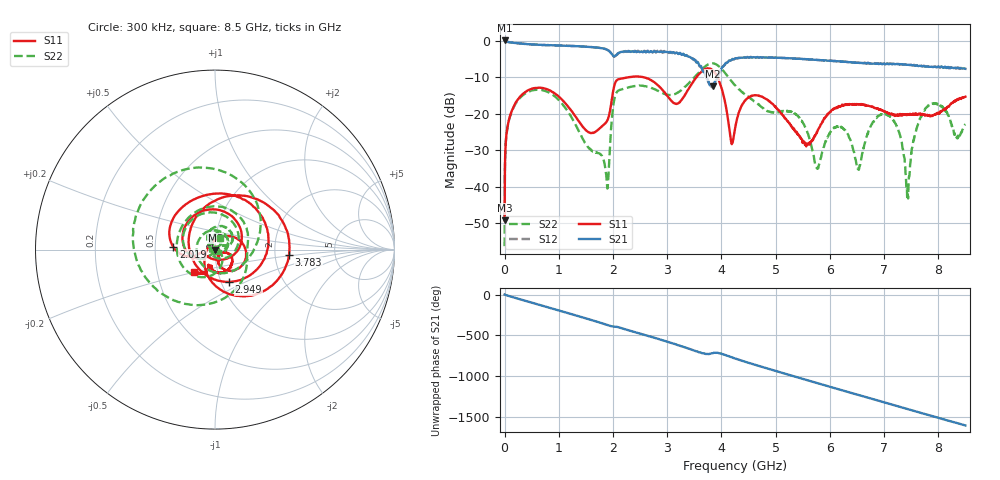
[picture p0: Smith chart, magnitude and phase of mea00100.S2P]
!Agilent Technologies,E5071B,MY42402595,A.08.01
!Date: Tue Jan 02 09:49:13 2001
!Data & Calibration Information:
!Freq	S11:SOLT2(ON)	S21:SOLT2(ON)	S12:SOLT2(ON)	S22:SOLT2(ON)
# Hz S dB R 50
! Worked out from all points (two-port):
!   1601 points, 300 kHz to 8.5 GHz, reference 50 ohm
!   highest |S21| = 0.03 dB at 300 kHz (marker M1); lowest = -12.5 dB at 3.841 GHz (marker M2)
!   |S21| within 3 dB of the highest: start of sweep to 1.937 GHz; 2.228 GHz to 2.254 GHz (25.67 MHz wide, 1.15 % of centre)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
!   lowest |S11| = -49.2 dB at 300 kHz (marker M3), VSWR 1.01, Z = 50.2 - j0.273 ohm
!   |S11| at or under -10 dB: start of sweep to 2.312 GHz; 2.55 GHz to 3.542 GHz (992 MHz wide, 32.6 % of centre); 3.925 GHz to end of sweep
!   |S22| runs from -56.3 to -6.2 dB; largest |S21 - S12| = 0.028
!   S11 on the Smith chart (normalised r, x): 300 kHz: 1.00, -0.01; 2.019 GHz: 0.62, +0.02; 2.949 GHz: 1.09, -0.41; 3.783 GHz: 2.40, -0.16; 8.5 GHz: 0.77, -0.20
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300000  -49.24 -52.1  0.03 0.2  0.00 -0.3  -56.32 -118.4
4.811081e7  -24.21 -137.5  -0.34 -11.0  -0.36 -11.1  -24.28 -137.5
1.490448e8  -18.68 -155.8  -0.58 -31.1  -0.59 -31.1  -18.84 -154.7
4.837204e8  -13.32 134.9  -1.03 -95.7  -1.05 -95.6  -13.77 140.8
8.5027e8  -13.79 59.2  -1.26 -165.2  -1.29 -165.2  -14.49 64.1
1.418687e9  -23.16 -54.0  -1.61 84.7  -1.61 84.7  -26.21 -75.5
1.886171e9  -22.13 -168.3  -2.49 -9.9  -2.49 -10.3  -38.99 106.3
2.018979e9  -12.64 176.2  -4.27 -30.3  -4.43 -30.7  -16.47 -101.2
2.428027e9  -9.83 53.6  -3.06 -104.3  -3.16 -103.9  -12.38 103.4
2.837075e9  -12.33 -36.3  -3.03 176.8  -3.03 175.1  -13.83 26.0
2.948633e9  -14.16 -66.7  -3.10 154.9  -2.92 153.7  -14.63 10.6
3.782666e9  -7.67 -3.9  -12.16 -5.1  -11.76 -4.1  -6.37 153.2
3.841102e9  -8.19 -24.6  -12.54 3.3  -12.16 5.8  -6.24 129.7
4.25015e9  -24.15 79.8  -4.94 -60.0  -4.96 -60.5  -12.26 11.9
4.850441e9  -16.25 -49.8  -4.67 176.2  -4.66 175.8  -19.33 -136.1
5.668537e9  -27.56 -27.0  -5.21 16.8  -5.21 16.8  -29.43 -42.1
6.258204e9  -17.72 -50.1  -5.77 -96.4  -5.84 -96.1  -24.24 60.9
6.529132e9  -17.46 -71.6  -6.10 -147.7  -6.04 -147.7  -35.36 80.2
7.086925e9  -19.86 -102.7  -6.51 107.3  -6.38 106.6  -20.65 43.4
7.432225e9  -20.13 -105.3  -6.63 40.6  -6.58 40.3  -43.31 -119.5
7.793462e9  -20.41 -113.4  -7.08 -27.7  -7.03 -27.7  -18.13 91.6
8.5e9  -15.38 -132.8  -7.74 -160.0  -7.70 -161.0  -22.96 65.4
